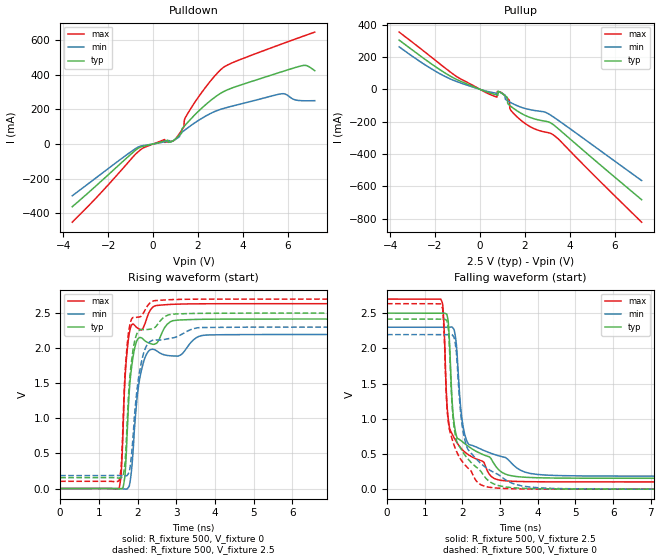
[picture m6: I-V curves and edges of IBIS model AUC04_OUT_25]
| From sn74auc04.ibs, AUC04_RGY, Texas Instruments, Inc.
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[Model]   AUC04_OUT_25
Model_type  Output
Vref =   0
Rref =   500
Cref =   30p
Vmeas =   1.25
| variable   typ   min   max
C_comp   3.5pF   NA   NA
| C_pullup   9.62pF   2.22pF   24.54pF
| C_pulldown   6.92pF   2.05pF   16.12pF
[Temperature Range]   40   100   -40
| Ambient temperature   25   85   -40
[Voltage range]   2.5   2.3   2.7
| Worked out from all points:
|   slope of the pulldown table from 0 to 0.375 V, typ, clamps not added: 30.7 ohm
|   slope of the pullup table from 0 to 0.375 V, typ, clamps not added: 19.1 ohm
|   rising waveform, R_fixture 500, V_fixture 0: 20-80 % time 194ps typ, 260ps min, 154ps max; typ from 0 V to 2.42 V
|   falling waveform, R_fixture 500, V_fixture 2.5: 20-80 % time 455ps typ, 462ps min, 382ps max; typ from 2.5 V to 0.155 V
|   rising waveform, R_fixture 500, V_fixture 2.5: 20-80 % time 196ps typ, 267ps min, 153ps max; typ from 0.154 V to 2.5 V
|   falling waveform, R_fixture 500, V_fixture 0: 20-80 % time 406ps typ, 485ps min, 329ps max; typ from 2.42 V to 0 V
[Pulldown]
| AUC04_OUT_25
|   Voltage   I(typ)   I(min)   I(max)
-3.6V     -363.3mA   -299.7mA   -452.8mA
-560mV    -17.97mA   -12.29mA   -33.51mA
510mV     17.07mA    12.84mA    25.87mA
975mV     26.82mA    25.47mA    25.82mA
1.27V     63.12mA    66.67mA    79.37mA
1.37V     100.7mA    76.6mA     99.34mA
1.42V     107.9mA    81.53mA    148.5mA
1.84V     166.6mA    121.2mA    238mA
3.1V      300.6mA    204.7mA    440.5mA
5.74V     418.9mA    291.2mA    579.9mA
6.745V    455.6mA    250.5mA    627.2mA
7.2V      424.9mA    251.1mA    648.3mA
[Pullup]
| AUC04_OUT_25
|   Voltage   I(typ)   I(min)   I(max)
-3.6V     305mA      263.2mA    354.5mA
-960mV    55.76mA    44.28mA    72.07mA
730mV     -33.82mA   -24.42mA   -47.21mA
760mV     -34.84mA   -25.13mA   -47.16mA
770mV     -35.18mA   -25.36mA   -13.25mA
980mV     -25.02mA   -24.81mA   -22.86mA
1.215V    -49.49mA   -69.56mA   -54.81mA
1.3V      -96.78mA   -76.45mA   -67.02mA
1.34V     -101.5mA   -79.57mA   -121.6mA
1.66V     -133.9mA   -101.4mA   -171.6mA
3.46V     -241mA     -189.3mA   -303.8mA
7.2V      -683.6mA   -565.1mA   -822.8mA
[Ramp]
| AUC04_OUT_25
| variable   typ   min   max
dV/dt_r   1.45/1.99E-10   1.32/2.63E-10   1.59/1.58E-10
dV/dt_f   1.41/4.56E-10   1.27/4.64E-10   1.56/3.83E-10
R_load = 500
[Rising Waveform]
| AUC04_OUT_25
R_fixture =   500
C_fixture =   0
L_fixture =   0
V_fixture =   0
V_fixture_min = 0
V_fixture_max = 0
|   Time   V(typ)   V(min)   V(max)
0s        13.01nV    39.01nV    2.017nV
1.52ns    -7.661mV   239.6uV    3.781mV
1.585ns   -1.006mV   -2.649mV   284.3mV
1.675ns   190.4mV    -7.776mV   1.558V
1.795ns   1.458V     60.88mV    2.238V
1.925ns   2V         888.6mV    2.325V
2.07ns    2.153V     1.608V     2.265V
2.475ns   2.066V     1.969V     2.607V
3.345ns   2.407V     2.061V     2.631V
22ns      2.416V     2.195V     2.634V
[Falling Waveform]
| AUC04_OUT_25
R_fixture =   500
C_fixture =   0
L_fixture =   0
V_fixture =   2.5
V_fixture_min = 2.3
V_fixture_max = 2.7
|   Time   V(typ)   V(min)   V(max)
0s        2.5V       2.3V       2.7V
1.425ns   2.499V     2.3V       2.699V
1.495ns   2.499V     2.299V     2.497V
1.595ns   2.467V     2.299V     1.177V
1.67ns    1.944V     2.301V     848.2mV
1.805ns   848.7mV    2.201V     705.8mV
1.97ns    686.6mV    1.083V     578.6mV
2.11ns    626.8mV    696.3mV    508.1mV
2.965ns   275.1mV    473.5mV    131mV
22ns      154.5mV    184.4mV    102.7mV
[Rising Waveform]
| AUC04_OUT_25
R_fixture =   500
C_fixture =   0
L_fixture =   0
V_fixture =   2.5
V_fixture_min = 2.3
V_fixture_max = 2.7
|   Time   V(typ)   V(min)   V(max)
0s        154.5mV    184.4mV    102.6mV
1.52ns    147.9mV    184.5mV    108.6mV
1.585ns   157.3mV    182.2mV    396.4mV
1.67ns    339.3mV    179.7mV    1.575V
1.795ns   1.555V     264.5mV    2.319V
1.92ns    2.089V     1.032V     2.441V
2.07ns    2.264V     1.72V      2.446V
2.425ns   2.285V     2.116V     2.676V
3.46ns    2.495V     2.28V      2.698V
22ns      2.5V       2.3V       2.7V
[Falling Waveform]
| AUC04_OUT_25
R_fixture =   500
C_fixture =   0
L_fixture =   0
V_fixture =   0
V_fixture_min = 0
V_fixture_max = 0
|   Time   V(typ)   V(min)   V(max)
0s        2.416V     2.195V     2.634V
1.43ns    2.414V     2.195V     2.627V
1.495ns   2.414V     2.195V     2.426V
1.59ns    2.389V     2.194V     1.176V
1.665ns   1.913V     2.194V     825.9mV
1.74ns    1.095V     2.186V     689.8mV
1.845ns   687.4mV    1.915V     536mV
2.08ns    475.4mV    668.2mV    337.9mV
2.63ns    151.8mV    305.3mV    36.09mV
22ns      50.77uV    16.49uV    23.37uV
